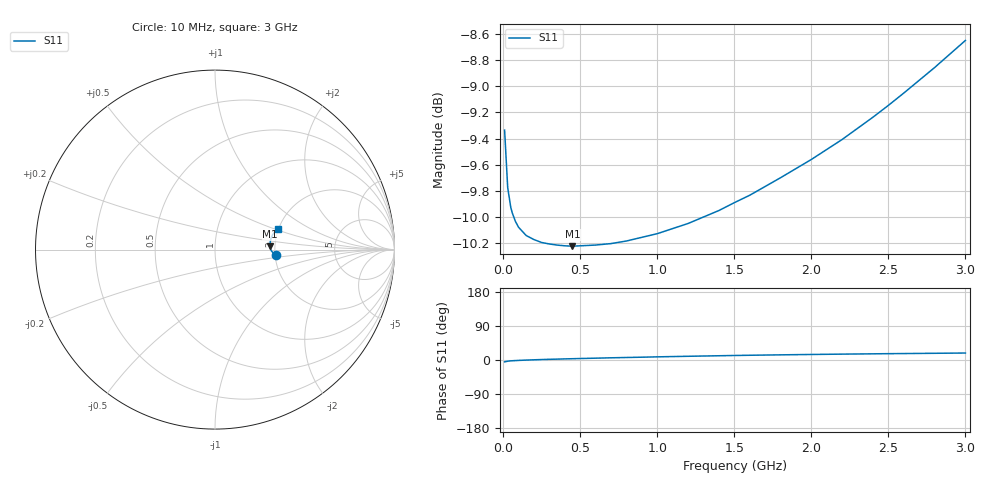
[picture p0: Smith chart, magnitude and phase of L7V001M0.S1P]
! SIEMENS Small Signal Semiconductors
! BAR14-1
! Si PIN Diode in SOT23
! IF = 1 mA
! S-Parameters:  July  1992
# GHz  S  MA  R  50
!  f  S11
! GHz  MAG  ANG
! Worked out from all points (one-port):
!   31 points, 10 MHz to 3 GHz, reference 50 ohm
!   lowest |S11| = -10.2 dB at 450 MHz (marker M1), VSWR 1.89, Z = 94.4 + j3.81 ohm
!   |S11| at or under -10 dB: 70.18 MHz to 1.296 GHz (1.226 GHz wide, 179 % of centre)
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0.01  0.3414 -4.8
0.03  0.3246 -3.2
0.05  0.319 -2.3
0.06  0.3174 -2.0
0.08  0.3151 -1.5
0.1  0.3135 -1.1
0.15  0.3112 -0.2
0.2  0.3101 0.5
0.25  0.3093 1.2
0.3  0.3089 1.8
0.35  0.3086 2.3
0.4  0.3084 2.9
0.45  0.3083 3.4
0.7  0.309 5.8
0.8  0.3097 6.6
0.9  0.3107 7.4
1  0.3117 8.3
1.2  0.3145 9.8
1.4  0.3181 11.2
1.5  0.3203 11.9
1.6  0.3224 12.5
2  0.3327 14.6
2.2  0.3386 15.5
2.4  0.3453 16.3
2.5  0.3489 16.7
2.6  0.3527 17.0
2.8  0.3607 17.7
3  0.3694 18.4
